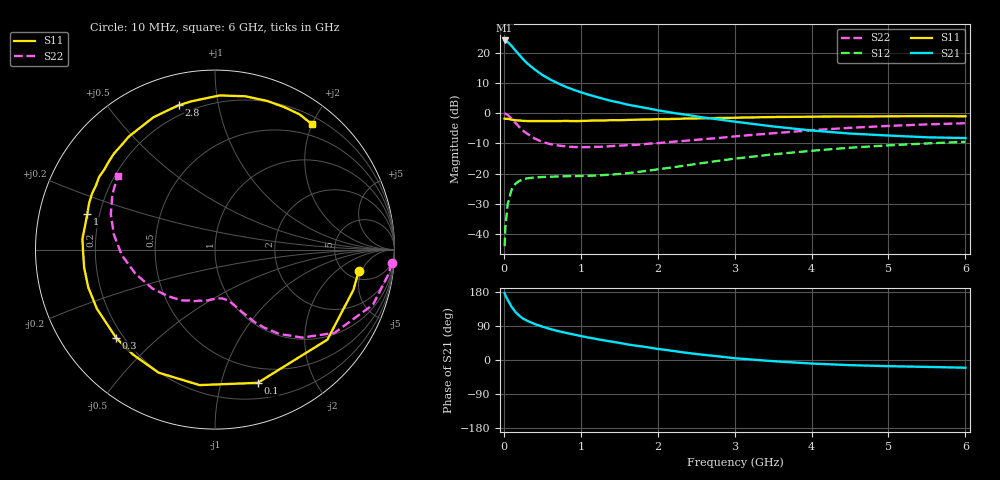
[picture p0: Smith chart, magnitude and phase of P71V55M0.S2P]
! SIEMENS Small Signal Semiconductors
! BFP196
! Si NPN RF Bipolar Junction Transistor in SOT143
! VCE = 1.5 V  IC = 5 mA
! Common Emitter S-Parameters:  May  1996
# GHz  S  MA  R  50
!  f  S11  S21  S12  S22
! GHz  MAG  ANG  MAG  ANG  MAG  ANG  MAG  ANG
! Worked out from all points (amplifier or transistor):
!   36 points, 10 MHz to 6 GHz, reference 50 ohm
!   highest |S21| = 24.0 dB at 10 MHz (marker M1)
!   |S21| within 3 dB of that: start of sweep to 140 MHz
!   unconditionally stable (mu >= 1): 1.111 GHz to 3.348 GHz; 5.609 GHz to end of sweep
!   at 250 MHz: K = 0.26, MSG = 19.9 dB, |S12| = -22.0 dB
!   at 1.4 GHz: K = 1.15, MAG = 9.8 dB, |S12| = -20.4 dB
!   at 6 GHz: K = 1.02, MAG = -0.3 dB, |S12| = -9.5 dB
!   S11 on the Smith chart (normalised r, x): 10 MHz: 6.43, -4.42; 100 MHz: 0.35, -1.31; 300 MHz: 0.17, -0.37; 1 GHz: 0.15, +0.13; 2.8 GHz: 0.15, +0.77; 6 GHz: 0.31, +2.00
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0.01  0.8098 -8.4  15.84 176.6  0.0063 87.0  0.9861 -4.2
0.02  0.8031 -16.3  15.45 170.9  0.0128 78.8  0.9769 -8.0
0.05  0.8024 -38.7  14.9 158.7  0.031 70.3  0.9324 -19.2
0.1  0.7797 -72.2  12.97 140.8  0.0538 55.1  0.8112 -34.9
0.15  0.7598 -96.5  10.81 127.0  0.0674 44.2  0.6895 -45.3
0.2  0.7543 -114.7  9.185 117.2  0.0754 36.6  0.5894 -52.8
0.25  0.7421 -128.1  7.752 109.4  0.0798 31.2  0.5105 -58.0
0.3  0.7382 -138.3  6.702 103.8  0.083 28.2  0.4581 -61.5
0.4  0.7359 -153.4  5.262 95.0  0.0863 23.6  0.3801 -66.5
0.5  0.7369 -163.4  4.263 88.0  0.0875 21.4  0.3336 -70.3
0.6  0.7359 -172.2  3.599 82.0  0.0888 20.4  0.3073 -73.3
0.7  0.7351 -178.9  3.116 76.6  0.0892 19.9  0.2919 -76.0
0.8  0.7409 175.3  2.733 71.9  0.0901 20.1  0.2814 -78.9
1  0.7386 164.4  2.206 63.3  0.091 21.9  0.2729 -84.8
1.1  0.7473 160.0  2.015 59.3  0.0919 23.1  0.274 -88.0
1.6  0.7678 140.7  1.385 41.5  0.1013 30.4  0.2942 -103.5
2.2  0.7979 121.1  1.006 23.9  0.1267 37.1  0.3356 -122.3
2.8  0.8293 104.0  0.782 9.4  0.163 37.2  0.3877 -142.3
3.5  0.8593 88.3  0.6 -3.1  0.2075 31.9  0.4634 -163.2
4.5  0.8779 70.7  0.458 -13.6  0.2673 20.6  0.5693 171.6
5.5  0.8887 58.0  0.397 -18.2  0.3146 8.3  0.6493 151.7
6  0.883 52.3  0.386 -20.4  0.3348 1.7  0.6791 143.0
